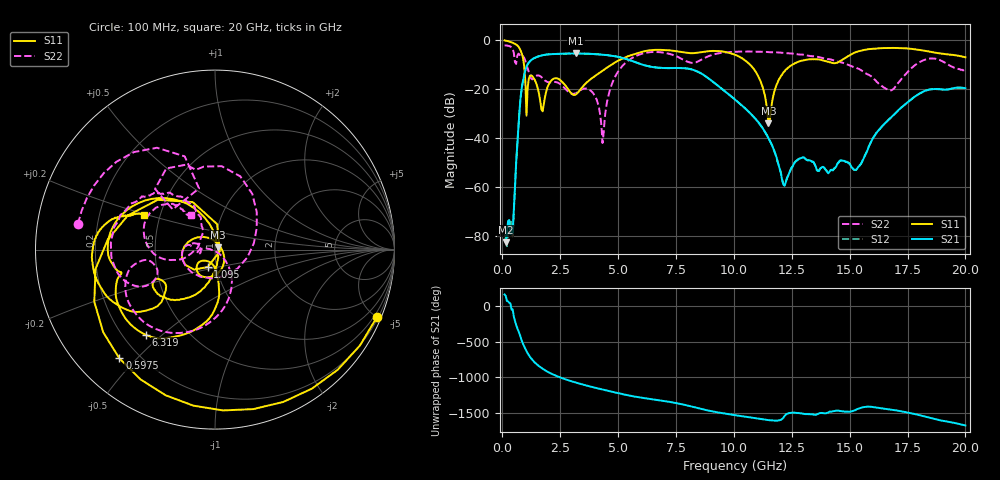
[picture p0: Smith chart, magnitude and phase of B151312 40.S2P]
!  2-Port S-parameters saved by WinCal
! VAR MeasName=S-Parameters (CALIBRATED_DATA) read from VNA (N5244A)
! VAR MeasDate=12/8/2015 5:46:47 PM
! VAR NAME=B151312 40
! VAR FILENAME=B151312 40.S2P
! VAR DATE=12/8/2015 5:46:47 PM
! VAR PHYS_PORTS=1,2
# Hz S DB R 50
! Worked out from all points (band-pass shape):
!   401 points, 100 MHz to 20 GHz, reference 50 ohm
!   highest |S21| = -5.51 dB at 3.184 GHz (marker M1); lowest = -82.7 dB at 149.8 MHz (marker M2)
!   |S21| within 3 dB of the highest: 1.216 GHz to 5.584 GHz (4.369 GHz wide, 128 % of centre)
!   lowest |S11| = -34.0 dB at 11.49 GHz (marker M3), VSWR 1.04, Z = 51.6 + j1.26 ohm
!   |S11| at or under -10 dB: 935.2 MHz to 4.73 GHz (3.795 GHz wide, 134 % of centre); 10.69 GHz to 12.54 GHz (1.852 GHz wide, 15.9 % of centre)
!   |S22| runs from -42.1 to -2.2 dB; largest |S21 - S12| = 0.0016
!   S11 on the Smith chart (normalised r, x): 100 MHz: 0.29, -4.99; 597.5 MHz: 0.13, -0.45; 1.095 GHz: 0.91, -0.18; 6.319 GHz: 0.29, -0.44; 20 GHz: 0.40, +0.20
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1e8  -0.20 -22.6  -81.59 158.4  -79.31 156.7  -2.19 169.3
1.4975e8  -0.28 -33.5  -82.69 138.6  -80.43 -157.1  -2.23 163.9
4.4825e8  -1.13 -97.9  -78.70 -49.5  -80.15 -54.5  -3.70 119.7
5.975e8  -1.86 -131.3  -50.17 94.8  -50.27 95.0  -9.76 136.4
8.4625e8  -5.65 158.6  -19.28 -132.6  -19.28 -132.7  -6.62 97.7
1.095e9  -19.59 -112.5  -9.94 55.3  -9.94 55.3  -11.66 27.2
1.493e9  -18.47 145.1  -6.93 -100.6  -6.93 -100.6  -14.52 -149.6
1.891e9  -21.26 -54.6  -5.98 168.2  -5.98 168.2  -16.85 169.6
2.43825e9  -15.97 -127.7  -5.67 84.4  -5.66 84.4  -17.62 165.1
3.1845e9  -22.20 -106.5  -5.51 3.4  -5.51 3.4  -21.78 -168.6
3.43325e9  -19.49 -89.0  -5.55 -19.5  -5.54 -19.5  -20.14 -165.5
4.32875e9  -12.54 -84.3  -5.99 -93.0  -5.99 -93.1  -42.07 -134.7
4.9755e9  -8.61 -93.5  -6.84 -141.8  -6.84 -141.8  -13.31 -64.5
6.31875e9  -4.28 -129.0  -10.73 137.8  -10.72 137.7  -5.03 -130.7
6.7665e9  -4.02 -142.2  -11.34 117.2  -11.34 117.1  -4.96 -148.1
1.005e10  -6.04 148.6  -24.31 -92.4  -24.32 -92.4  -4.78 -174.4
1.149275e10  -34.04 37.9  -40.02 -161.9  -40.05 -161.9  -4.95 164.5
1.218925e10  -12.80 -107.4  -59.53 -105.1  -59.24 -104.4  -5.35 154.5
1.338325e10  -7.85 -144.6  -49.76 -80.5  -49.66 -81.4  -6.66 138.0
1.527375e10  -4.94 -142.2  -53.08 -15.2  -53.08 -14.8  -11.39 115.7
1.67165e10  -3.28 -172.1  -32.29 -11.9  -32.22 -13.0  -20.58 158.4
2e10  -7.07 153.9  -19.72 123.4  -19.78 123.1  -12.60 125.3
